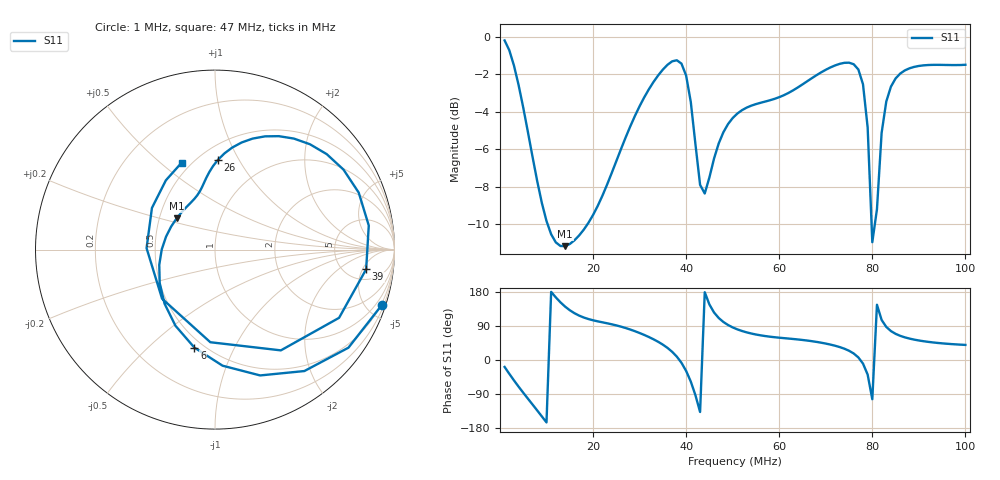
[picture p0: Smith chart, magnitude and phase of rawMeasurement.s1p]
# MHz S RI R 50.0
! SimSmith 18.4f
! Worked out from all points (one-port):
!   100 points, 1 MHz to 100 MHz, reference 50 ohm
!   lowest |S11| = -11.2 dB at 14 MHz (marker M1), VSWR 1.76, Z = 30.7 + j11.6 ohm
!   |S11| at or under -10 dB: 10.22 MHz to 18.85 MHz (8.636 MHz wide, 59.4 % of centre); 79.84 MHz to 80.56 MHz (715.1 kHz wide, 0.892 % of centre)
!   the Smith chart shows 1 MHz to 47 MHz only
!   S11 on the Smith chart (normalised r, x): 1 MHz: 0.40, -6.17; 6 MHz: 0.45, -0.71; 26 MHz: 0.62, +0.82; 39 MHz: 7.56, -5.93; 47 MHz: 0.45, +0.59
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1  0.9299 -0.3083
3  0.4979 -0.6766
6  -0.1151 -0.5457
9  -0.3081 -0.186
14  -0.2139 0.1739
26  0.0171 0.501
31  0.279 0.631
34  0.5289 0.587
37  0.8007 0.3175
39  0.8422 -0.1094
40  0.6913 -0.38
41  0.3669 -0.5614
42  -0.0261 -0.5161
43  -0.295 -0.2734
44  -0.3813 0.00808
47  -0.1851 0.4852
51  0.0991 0.6164
63  0.4088 0.5933
71  0.6289 0.5409
76  0.8082 0.2503
78  0.7379 -0.123
79  0.449 -0.356
80  -0.0668 -0.2744
81  -0.2862 0.1947
82  -0.1505 0.5332
83  0.0319 0.6714
88  0.4558 0.6879
100  0.6479 0.5397
